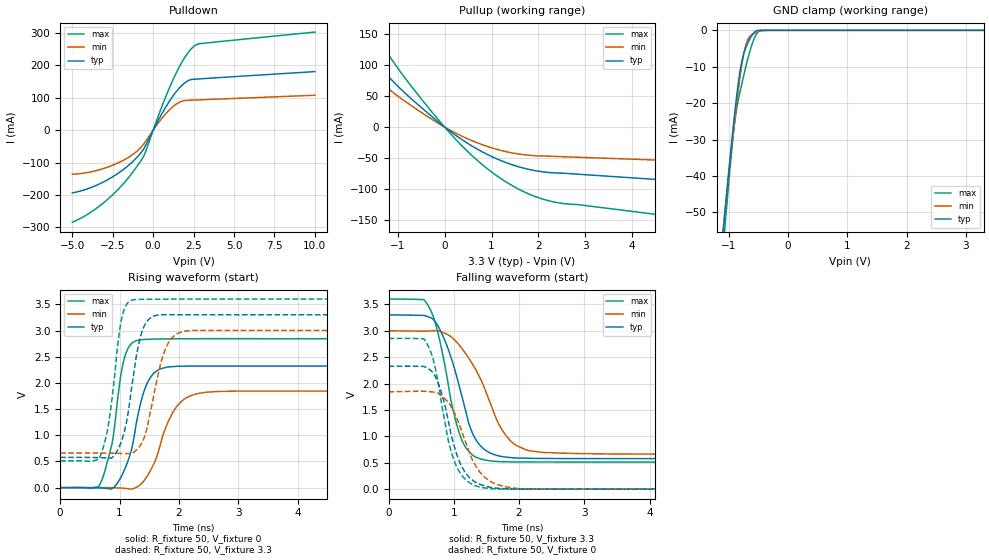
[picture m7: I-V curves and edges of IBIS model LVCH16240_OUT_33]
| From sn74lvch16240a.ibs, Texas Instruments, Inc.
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[Model]   LVCH16240_OUT_33
Model_type  3-state
Enable   Active-Low
Vref =   0
Rref =   500
Cref =   50p
Vmeas =   1.5
| variable   typ   min   max
C_comp   4.64pF   4.12pF   5.98pF
| C_pullup   6.54pF   3.89pF   9.70pF
| C_pulldown   6.88pF   5.28pF   8.79pF
| C_tri-state   4.64pF   4.12pF   5.98pF
[Temperature Range]   40   100   -40
| Ambient temperature   25   85   -40
[Voltage range]   3.3   3   3.6
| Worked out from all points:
|   slope of the pulldown table from 0 to 0.495 V, typ, clamps not added: 10.5 ohm
|   slope of the pullup table from 0 to 0.495 V, typ, clamps not added: 18.7 ohm
|   GND clamp passes 1 mA (typ) near -0.59 V on its own axis
|   rising waveform, R_fixture 50, V_fixture 0: 20-80 % time 291ps typ, 378ps min, 229ps max; typ from 0 V to 2.32 V
|   falling waveform, R_fixture 50, V_fixture 3.3: 20-80 % time 383ps typ, 535ps min, 315ps max; typ from 3.3 V to 0.578 V
|   rising waveform, R_fixture 50, V_fixture 3.3: 20-80 % time 234ps typ, 276ps min, 198ps max; typ from 0.578 V to 3.3 V
|   falling waveform, R_fixture 50, V_fixture 0: 20-80 % time 304ps typ, 375ps min, 279ps max; typ from 2.33 V to 0 V
[GND Clamp]
| LVCH16240_OUT_33
|   Voltage   I(typ)   I(min)   I(max)
-5V       -855.7mA   -797.6mA   -953.2mA
-1.095V   -55.25mA   -54.79mA   -60.22mA
-1.065V   -49.94mA   -49.9mA    -54.27mA
-955mV    -31.29mA   -32.66mA   -33.81mA
-910mV    -24.24mA   -26.03mA   -26.76mA
-860mV    -17.12mA   -19.11mA   -20.92mA
-795mV    -9.817mA   -11.17mA   -15.81mA
-735mV    -5.784mA   -5.591mA   -11.55mA
-680mV    -3.534mA   -2.583mA   -7.881mA
-580mV    -736.5uA   -852.5uA   -2.652mA
-485mV    -14.03uA   -258.5uA   -126.7uA
3.3V      10.95pA    56.13nA    -148.6pA
[Pulldown]
| LVCH16240_OUT_33
|   Voltage   I(typ)   I(min)   I(max)
-5V       -193.4mA   -135.8mA   -283.8mA
-3.87V    -177.4mA   -128.6mA   -253.7mA
-2.72V    -150.1mA   -112.1mA   -209.2mA
-1.54V    -109.1mA   -84.13mA   -147.4mA
-730mV    -67.77mA   -51.47mA   -92.05mA
-485mV    -48.43mA   -35.35mA   -68.52mA
485mV     46.17mA    33.18mA    66.28mA
1.245V    107.2mA    73.64mA    157.8mA
1.945V    145.9mA    91.78mA    224mA
2.535V    157.6mA    93.17mA    259.6mA
2.87V     158.7mA    93.86mA    267.5mA
10V       181.2mA    108.1mA    303.1mA
[Pullup]
| LVCH16240_OUT_33
|   Voltage   I(typ)   I(min)   I(max)
-5V       388.2mA    115.6mA    569.5mA
-4.8V     377.1mA    131.8mA    547.8mA
-4.67V    368.8mA    170.1mA    533.4mA
-2.73V    213.4mA    164.5mA    302.6mA
-2.425V   186.8mA    144.1mA    265.2mA
-1.63V    117.9mA    90.44mA    167.3mA
-735mV    47.21mA    35.83mA    68.13mA
480mV     -25.67mA   -18.52mA   -38.57mA
1.275V    -56.24mA   -38.95mA   -86.83mA
2.13V     -72.49mA   -46.66mA   -117mA
6.525V    -94.6mA    -58.57mA   -160mA
10V       -112.3mA   -68.03mA   -193.4mA
[Ramp]
| LVCH16240_OUT_33
| variable   typ   min   max
dV/dt_r   1.41/2.97E-10   1.12/3.99E-10   1.71/2.34E-10
dV/dt_f   1.63/4.01E-10   1.41/5.57E-10   1.85/3.27E-10
R_load = 50
[Rising Waveform]
| LVCH16240_OUT_33
R_fixture =   50
C_fixture =   0
L_fixture =   0
V_fixture =   0
V_fixture_min = 0
V_fixture_max = 0
|   Time   V(typ)   V(min)   V(max)
0s        353.3uV    56.06uV    564.8uV
660ps     -4.389mV   2.153mV    44.93mV
875ps     -17.59mV   -1.395mV   849.1mV
1.01ns    173.6mV    -6.534mV   2.067V
1.095ns   375.9mV    -14.45mV   2.527V
1.455ns   1.97V      204.3mV    2.831V
1.655ns   2.248V     697.9mV    2.838V
1.98ns    2.317V     1.575V     2.842V
2.69ns    2.321V     1.838V     2.844V
50ns      2.322V     1.845V     2.844V
[Falling Waveform]
| LVCH16240_OUT_33
R_fixture =   50
C_fixture =   0
L_fixture =   0
V_fixture =   3.3
V_fixture_min = 3
V_fixture_max = 3.6
|   Time   V(typ)   V(min)   V(max)
0s        3.299V     2.998V     3.599V
540ps     3.29V      2.99V      3.589V
705ps     3.188V     3.001V     3.195V
920ps     2.632V     2.916V     1.953V
1.14ns    1.685V     2.639V     883.6mV
1.345ns   924.2mV    2.245V     601mV
1.71ns    622.9mV    1.188V     520.7mV
2.145ns   584.3mV    731mV      514.1mV
3.41ns    577.2mV    665.4mV    512.5mV
50ns      578.1mV    661.9mV    513mV
[Rising Waveform]
| LVCH16240_OUT_33
R_fixture =   50
C_fixture =   0
L_fixture =   0
V_fixture =   3.3
V_fixture_min = 3
V_fixture_max = 3.6
|   Time   V(typ)   V(min)   V(max)
0s        578.1mV    661.8mV    513mV
665ps     573.1mV    661.2mV    580.9mV
815ps     565.6mV    659.2mV    1.229V
1.03ns    876.4mV    653.6mV    3.199V
1.13ns    1.336V     650.4mV    3.516V
1.28ns    2.498V     715.4mV    3.593V
1.46ns    3.174V     1.136V     3.595V
1.8ns     3.303V     2.719V     3.599V
2.235ns   3.299V     3.001V     3.6V
50ns      3.299V     2.998V     3.599V
[Falling Waveform]
| LVCH16240_OUT_33
R_fixture =   50
C_fixture =   0
L_fixture =   0
V_fixture =   0
V_fixture_min = 0
V_fixture_max = 0
|   Time   V(typ)   V(min)   V(max)
0s        2.326V     1.843V     2.853V
555ps     2.317V     1.852V     2.824V
680ps     2.211V     1.839V     2.479V
775ps     1.959V     1.801V     1.916V
910ps     1.331V     1.648V     956.7mV
1.04ns    680mV      1.361V     435.5mV
1.325ns   136.9mV    462.4mV    67.16mV
1.605ns   26.34mV    118.9mV    7.492mV
2.32ns    574.9uV    -1.335mV   347.1uV
50ns      336.9uV    99.47uV    530uV
